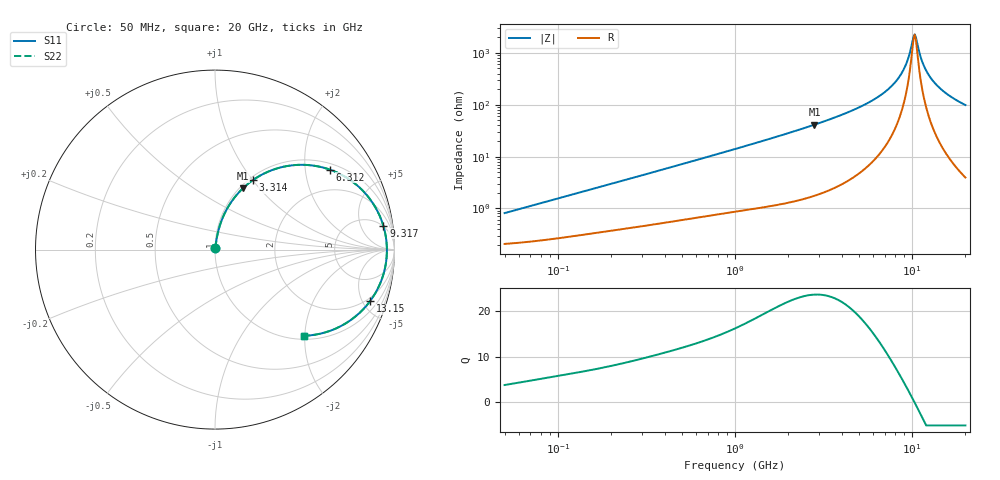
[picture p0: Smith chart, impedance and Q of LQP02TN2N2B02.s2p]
!Murata Part Number: LQP02TN2N2B02
!These Parameters are Measured in Series Mode Connection
!  o--[Z]--o
!Port1  Port2
!  o-------o
!Freq. Start=50[MHz] Stop=20[GHz], 401[Steps]
# Hz S RI R 50
!Freq.(Hz) S11(Real) S11(Imag) S21(Real) S21(Imag) S12(Real) S12(Imag) S22(Real) S22(Imag)
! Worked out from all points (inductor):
!   401 points, 50 MHz to 20 GHz, reference 50 ohm
!   read as one part in series: L = 2.49 nH near 51.52 MHz
!   highest Q = 23.5 at 2.811 GHz (marker M1), where L = 2.33 nH
!   self-resonance near 10.33 GHz
!   S11 on the Smith chart (normalised r, x): 50 MHz: 1.00, +0.02; 3.314 GHz: 1.04, +1.00; 6.312 GHz: 1.19, +2.72; 9.317 GHz: 5, +12; 13.15 GHz: 1.69, -5.68; 20 GHz: 1.08, -1.97
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5e7  0.00213 0.00784  0.9979 -0.00784  0.9979 -0.00784  0.00213 0.00784
1.364002e8  0.00349 0.0205  0.9965 -0.0205  0.9965 -0.0205  0.00349 0.0205
3.721004e8  0.00788 0.0528  0.9921 -0.0528  0.9921 -0.0528  0.00788 0.0528
1e9  0.0272 0.1346  0.9728 -0.1346  0.9728 -0.1346  0.0272 0.1346
1.793498e9  0.0697 0.232  0.9303 -0.232  0.9303 -0.232  0.0697 0.232
2.728004e9  0.1475 0.3339  0.8525 -0.3339  0.8525 -0.3339  0.1475 0.3339
2.810964e9  0.1558 0.342  0.8442 -0.342  0.8442 -0.342  0.1558 0.342
3.314454e9  0.211 0.387  0.789 -0.387  0.789 -0.387  0.211 0.387
4.539627e9  0.3735 0.4598  0.6265 -0.4598  0.6265 -0.4598  0.3735 0.4598
6.311513e9  0.64 0.4456  0.36 -0.4456  0.36 -0.4456  0.64 0.4456
7.442007e9  0.7899 0.3596  0.2101 -0.3596  0.2101 -0.3596  0.7899 0.3596
8.516016e9  0.8925 0.2373  0.1075 -0.2373  0.1075 -0.2373  0.8925 0.2373
9.316812e9  0.9378 0.1331  0.0622 -0.1331  0.0622 -0.1331  0.9378 0.1331
1.004137e10  0.956 0.0377  0.044 -0.0377  0.044 -0.0377  0.956 0.0377
1.034674e10  0.9577 -0.00147  0.0423 0.00147  0.0423 0.00147  0.9577 -0.00147
1.066139e10  0.9563 -0.0407  0.0437 0.0407  0.0437 0.0407  0.9563 -0.0407
1.115139e10  0.9481 -0.0987  0.0519 0.0987  0.0519 0.0987  0.9481 -0.0987
1.166392e10  0.933 -0.1549  0.067 0.1549  0.067 0.1549  0.933 -0.1549
1.238412e10  0.9031 -0.225  0.0969 0.225  0.0969 0.225  0.9031 -0.225
1.314879e10  0.8636 -0.2877  0.1364 0.2877  0.1364 0.2877  0.8636 -0.2877
1.573793e10  0.7098 -0.4216  0.2902 0.4216  0.2902 0.4216  0.7098 -0.4216
2e10  0.4934 -0.4804  0.5066 0.4804  0.5066 0.4804  0.4934 -0.4804
